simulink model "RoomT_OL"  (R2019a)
settings: Solver=ode15s  StartTime=0.0  StopTime=tend  RelTol=1e-3
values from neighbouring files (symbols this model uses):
  m_in0 = 0.4    [mainOL.m]    (also in mainV3.m; mainV3_SRC.m)
  m_in_1 = 0    [mainOL.m]
  m_in_2 = 0    [mainOL.m]
  p = [m,Cp, Ufl, Afl, mfl, Cpfl]'    [mainOL.m]    (also in mainV3.m; mainV3_SRC.m)
  QAC0 = 0    [mainOL.m]    (also in mainV3.m; mainV3_SRC.m)
  QAC_1 = 0    [mainOL.m]
  QAC_2 = 0    [mainOL.m]
  QH10 = 0    [mainOL.m]    (also in mainV3.m; mainV3_SRC.m)
  QH1_1 = 0    [mainOL.m]
  QH1_2 = 0    [mainOL.m]
  QH20 = 0    [mainOL.m]    (also in mainV3.m; mainV3_SRC.m)
  QH2_1 = 1    [mainOL.m]
  QH2_2 = 0    [mainOL.m]
  Tin0 = 21    [mainOL.m]    (also in mainV3.m; mainV3_SRC.m)
  Tin_1 = 0    [mainOL.m]    (also in mainV3.m = 10; mainV3_SRC.m = 10)
  Tin_2 = 0    [mainOL.m]    (also in mainV3.m = -5; mainV3_SRC.m = -5)
  tm_in_1 = 40000    [mainOL.m]
  tm_in_2 = 2    [mainOL.m]
  tQAC_1 = 10    [mainOL.m]
  tQAC_2 = 140000    [mainOL.m]
  tQH1_1 = 10    [mainOL.m]
  tQH1_2 = 65000    [mainOL.m]
  tQH2_1 = 10    [mainOL.m]
  tQH2_2 = 40000    [mainOL.m]
  tTin_1 = 190000    [mainOL.m]    (also in mainV3.m = 1800; mainV3_SRC.m = 1800)
  tTin_2 = 2    [mainOL.m]    (also in mainV3.m = 12600; mainV3_SRC.m = 12600)
  x0 = [T0; Tfl0]    [mainOL.m]    (also in mainV3.m; mainV3_SRC.m; col_obj.m = 0.5*ones(1,82)'; Simulate1Col.m = x)
undefined symbols (not defined in the file or in its folder): Room

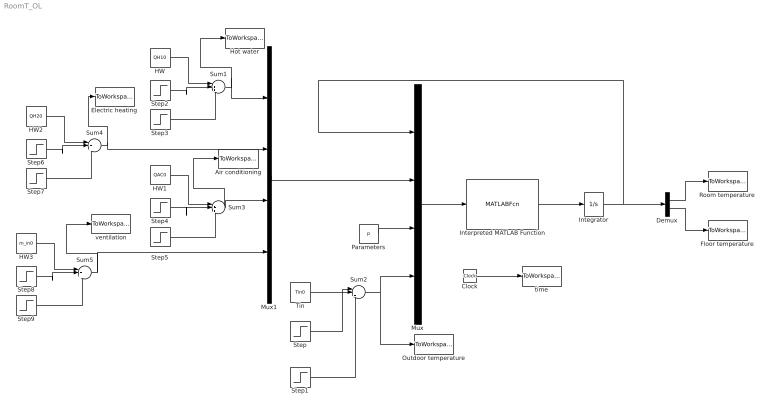
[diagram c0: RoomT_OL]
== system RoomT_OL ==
  Air conditioning : ToWorkspace  VariableName=QAC  SampleTime=-1
  Clock : Clock
  Demux : Demux  Outputs=2
  Electric heating : ToWorkspace  VariableName=QH2  SampleTime=-1
  Floor temperature : ToWorkspace  VariableName=Tfl  SampleTime=-1
  HW : Constant  Value=QH10
  HW1 : Constant  Value=QAC0
  HW2 : Constant  Value=QH20
  HW3 : Constant  Value=m_in0
  Hot water : ToWorkspace  VariableName=QH1  SampleTime=-1
  Integrator : Integrator  InitialCondition=x0'
  Interpreted MATLAB Function : MATLABFcn  MATLABFcn=Room(u)  OutputDimensions=2  Output1D=off
  Mux : Mux
  Mux1 : Mux
  Outdoor temperature : ToWorkspace  VariableName=Tin  SampleTime=-1
  Parameters : Constant  Value=p
  Room temperature : ToWorkspace  VariableName=T  SampleTime=-1
  Step : Step  Time=tTin_1  After=Tin_1  SampleTime=0
  Step1 : Step  Time=tTin_2  After=Tin_2  SampleTime=0
  Step2 : Step  Time=tQH1_1  After=QH1_1  SampleTime=0
  Step3 : Step  Time=tQH1_2  After=QH1_2  SampleTime=0
  Step4 : Step  Time=tQAC_1  After=QAC_1  SampleTime=0
  Step5 : Step  Time=tQAC_2  After=QAC_2  SampleTime=0
  Step6 : Step  Time=tQH2_1  After=QH2_1  SampleTime=0
  Step7 : Step  Time=tQH2_2  After=QH2_2  SampleTime=0
  Step8 : Step  Time=tm_in_1  After=m_in_1  SampleTime=0
  Step9 : Step  Time=tm_in_2  After=m_in_2  SampleTime=0
  Sum{1..5} (5 alike) : Sum  Inputs=|+++
  Tin : Constant  Value=Tin0
  time : ToWorkspace  VariableName=t  SampleTime=-1
  ventilation : ToWorkspace  VariableName=m_in  SampleTime=-1
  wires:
  Clock/1 -> time/1
  Interpreted MATLAB Function/1 -> Integrator/1
  Mux/1 -> Interpreted MATLAB Function/1
  Integrator/1 -> Demux/1, Mux/1
  Parameters/1 -> Mux/3
  Sum2/1 -> Outdoor temperature/1, Mux/4
  Step1/1 -> Sum2/3
  Step/1 -> Sum2/2
  Tin/1 -> Sum2/1
  Mux1/1 -> Mux/2
  Step3/1 -> Sum1/3
  Sum1/1 -> Hot water/1, Mux1/1
  Step2/1 -> Sum1/2
  HW/1 -> Sum1/1
  HW1/1 -> Sum3/1
  Sum3/1 -> Air conditioning/1, Mux1/3
  Step5/1 -> Sum3/3
  Step4/1 -> Sum3/2
  HW2/1 -> Sum4/1
  Sum4/1 -> Mux1/2, Electric heating/1
  Step7/1 -> Sum4/3
  Step6/1 -> Sum4/2
  HW3/1 -> Sum5/1
  Sum5/1 -> Mux1/4, ventilation/1
  Step9/1 -> Sum5/3
  Step8/1 -> Sum5/2
  Demux/1 -> Room temperature/1
  Demux/2 -> Floor temperature/1
